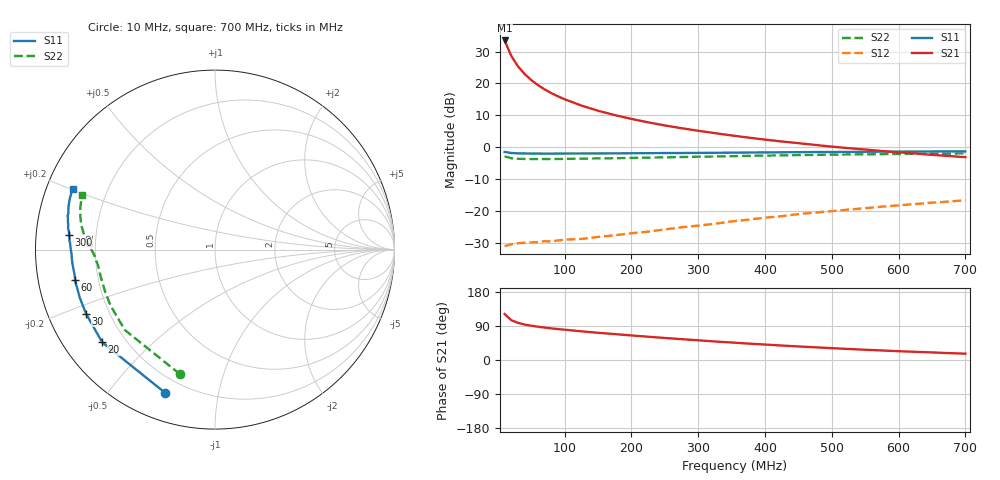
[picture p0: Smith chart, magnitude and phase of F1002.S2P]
! Date: Mon Aug 07 13:19:40 1995
# MHZ  S  MA  R  50.0000
!  POLYFET RF DEVICES
!  F1002
!  S PARAMETERS
!  VDS=28V, IDQ=400mA
!FREQ  S11MAG S11ANG S21MAG S21ANG S12MAG S12ANG S22MAG S22ANG
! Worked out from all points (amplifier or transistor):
!   34 points, 10 MHz to 700 MHz, reference 50 ohm
!   highest |S21| = 33.5 dB at 10 MHz (marker M1)
!   |S21| within 3 dB of that: start of sweep to 16.19 MHz
!   unconditionally stable (mu >= 1): 207.3 MHz to 371.2 MHz
!   at 60 MHz: K = 0.43, MSG = 24.6 dB, |S12| = -29.7 dB
!   at 300 MHz: K = 1.05, MAG = 13.5 dB, |S12| = -24.6 dB
!   at 700 MHz: K = 0.77, MSG = 6.7 dB, |S12| = -16.6 dB
!   S11 on the Smith chart (normalised r, x): 10 MHz: 0.13, -0.71; 20 MHz: 0.12, -0.35; 30 MHz: 0.12, -0.23; 60 MHz: 0.11, -0.11; 300 MHz: 0.10, +0.05; 700 MHz: 0.08, +0.20
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10  0.8458 -109.0  47.21 121.4  0.02818 37.1  0.7212 -105.7
20  0.8135 -140.6  27.03 105.0  0.03013 23.5  0.673 -138.2
30  0.8023 -153.6  18.54 98.0  0.03132 20.2  0.6605 -151.5
40  0.7998 -160.4  14.04 93.6  0.03192 19.1  0.6558 -158.6
50  0.7973 -164.7  11.28 90.4  0.03221 20.5  0.654 -163.0
60  0.798 -167.7  9.414 87.9  0.03264 21.4  0.6543 -166.1
70  0.7946 -169.9  8.074 85.6  0.03376 23.9  0.6545 -168.3
80  0.7954 -171.4  7.055 83.5  0.03341 24.0  0.654 -169.9
90  0.7968 -172.9  6.278 81.6  0.03465 26.2  0.6561 -171.2
100  0.7979 -174.1  5.647 79.9  0.03569 28.1  0.6574 -172.3
125  0.7993 -176.4  4.501 75.7  0.03656 32.1  0.6635 -174.4
150  0.7994 -178.2  3.735 71.8  0.03935 35.7  0.6685 -176.1
175  0.8027 -179.7  3.19 68.4  0.04177 39.6  0.6743 -177.5
200  0.806 178.8  2.782 64.8  0.04492 43.7  0.6805 -178.7
225  0.8076 177.6  2.459 61.4  0.04761 46.2  0.6876 -179.8
250  0.8127 176.5  2.197 58.1  0.0516 49.3  0.6955 179.1
300  0.817 174.3  1.812 52.0  0.05921 52.8  0.711 176.9
375  0.8275 171.6  1.419 43.3  0.07334 55.6  0.733 173.6
425  0.8342 169.3  1.233 38.2  0.08329 57.0  0.7465 171.3
475  0.8422 167.1  1.089 33.5  0.09485 56.5  0.7595 168.9
600  0.8548 161.8  0.8332 23.2  0.123 54.2  0.7857 162.7
700  0.8603 156.8  0.6988 16.7  0.1478 50.6  0.7985 157.8
